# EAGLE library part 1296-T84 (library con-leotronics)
1.27mm SINGLE ROW FEMALE SOCKET Source: http://www.leotronics.co.uk/Conexcon/Data%20Sheets/sec.%20A/1296ing.pdf
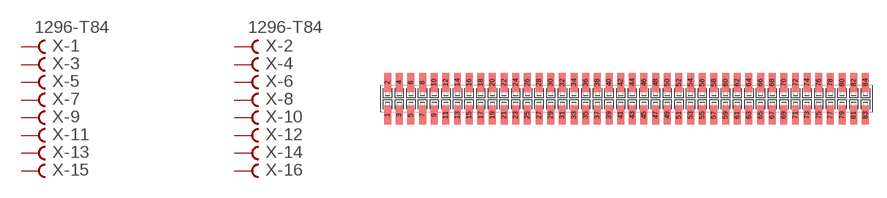
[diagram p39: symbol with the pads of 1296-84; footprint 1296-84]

Designator prefix X; gates -1=FVAL -2=FVAL -3=F -4=F -5=F -6=F -7=F -8=F -9=F -10=F -11=F -12=F -13=F -14=F -15=F -16=F -17=F -18=F -19=F -20=F -21=F -22=F -23=F -24=F -25=F -26=F -27=F -28=F -29=F -30=F -31=F -32=F -33=F -34=F -35=F -36=F -37=F -38=F -39=F -40=F -41=F -42=F -43=F -44=F -45=F -46=F -47=F -48=F -49=F -50=F -51=F -52=F -53=F -54=F -55=F -56=F -57=F -58=F -59=F -60=F -61=F -62=F -63=F -64=F -65=F -66=F -67=F -68=F -69=F -70=F -71=F -72=F -73=F -74=F -75=F -76=F -77=F -78=F -79=F -80=F -81=F -82=F -83=F -84=F

## 1296-T84 (OC_FARNELL: unknown; OC_NEWARK: unknown)  [1296-84]
1  -1:B  pas
2  -2:B  pas
3  -3:B  pas
4  -4:B  pas
5  -5:B  pas
6  -6:B  pas
7  -7:B  pas
8  -8:B  pas
9  -9:B  pas
10  -10:B  pas
11  -11:B  pas
12  -12:B  pas
13  -13:B  pas
14  -14:B  pas
15  -15:B  pas
16  -16:B  pas
17  -17:B  pas
18  -18:B  pas
19  -19:B  pas
20  -20:B  pas
21  -21:B  pas
22  -22:B  pas
23  -23:B  pas
24  -24:B  pas
25  -25:B  pas
26  -26:B  pas
27  -27:B  pas
28  -28:B  pas
29  -29:B  pas
30  -30:B  pas
31  -31:B  pas
32  -32:B  pas
33  -33:B  pas
34  -34:B  pas
35  -35:B  pas
36  -36:B  pas
37  -37:B  pas
38  -38:B  pas
39  -39:B  pas
40  -40:B  pas
41  -41:B  pas
42  -42:B  pas
43  -43:B  pas
44  -44:B  pas
45  -45:B  pas
46  -46:B  pas
47  -47:B  pas
48  -48:B  pas
49  -49:B  pas
50  -50:B  pas
51  -51:B  pas
52  -52:B  pas
53  -53:B  pas
54  -54:B  pas
55  -55:B  pas
56  -56:B  pas
57  -57:B  pas
58  -58:B  pas
59  -59:B  pas
60  -60:B  pas
61  -61:B  pas
62  -62:B  pas
63  -63:B  pas
64  -64:B  pas
65  -65:B  pas
66  -66:B  pas
67  -67:B  pas
68  -68:B  pas
69  -69:B  pas
70  -70:B  pas
71  -71:B  pas
72  -72:B  pas
73  -73:B  pas
74  -74:B  pas
75  -75:B  pas
76  -76:B  pas
77  -77:B  pas
78  -78:B  pas
79  -79:B  pas
80  -80:B  pas
81  -81:B  pas
82  -82:B  pas
83  -83:B  pas
84  -84:B  pas

## Footprint 1296-84 (pad centres in mm)
1.27mm SINGLE ROW FEMALE SOCKET Source: http://www.leotronics.co.uk/Conexcon/Data%20Sheets/sec.%20A/1296ing.pdf
smd 0.76 x 2.05: 1 -26.035,-1.78; 2 -26.035,1.78; 3 -24.765,-1.78; 4 -24.765,1.78; 5 -23.495,-1.78; 6 -23.495,1.78; 7 -22.225,-1.78; 8 -22.225,1.78; 9 -20.955,-1.78; 10 -20.955,1.78; 11 -19.685,-1.78; 12 -19.685,1.78; 13 -18.415,-1.78; 14 -18.415,1.78; 15 -17.145,-1.78; 16 -17.145,1.78; 17 -15.875,-1.78; 18 -15.875,1.78; 19 -14.605,-1.78; 20 -14.605,1.78; 21 -13.335,-1.78; 22 -13.335,1.78; 23 -12.065,-1.78; 24 -12.065,1.78; 25 -10.795,-1.78; 26 -10.795,1.78; 27 -9.525,-1.78; 28 -9.525,1.78; 29 -8.255,-1.78; 30 -8.255,1.78; 31 -6.985,-1.78; 32 -6.985,1.78; 33 -5.715,-1.78; 34 -5.715,1.78; 35 -4.445,-1.78; 36 -4.445,1.78; 37 -3.175,-1.78; 38 -3.175,1.78; 39 -1.905,-1.78; 40 -1.905,1.78; 41 -0.635,-1.78; 42 -0.635,1.78; 43 0.635,-1.78; 44 0.635,1.78; 45 1.905,-1.78; 46 1.905,1.78; 47 3.175,-1.78; 48 3.175,1.78; 49 4.445,-1.78; 50 4.445,1.78; 51 5.715,-1.78; 52 5.715,1.78; 53 6.985,-1.78; 54 6.985,1.78; 55 8.255,-1.78; 56 8.255,1.78; 57 9.525,-1.78; 58 9.525,1.78; 59 10.795,-1.78; 60 10.795,1.78; 61 12.065,-1.78; 62 12.065,1.78; 63 13.335,-1.78; 64 13.335,1.78; 65 14.605,-1.78; 66 14.605,1.78; 67 15.875,-1.78; 68 15.875,1.78; 69 17.145,-1.78; 70 17.145,1.78; 71 18.415,-1.78; 72 18.415,1.78; 73 19.685,-1.78; 74 19.685,1.78; 75 20.955,-1.78; 76 20.955,1.78; 77 22.225,-1.78; 78 22.225,1.78; 79 23.495,-1.78; 80 23.495,1.78; 81 24.765,-1.78; 82 24.765,1.78; 83 26.035,-1.78; 84 26.035,1.78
